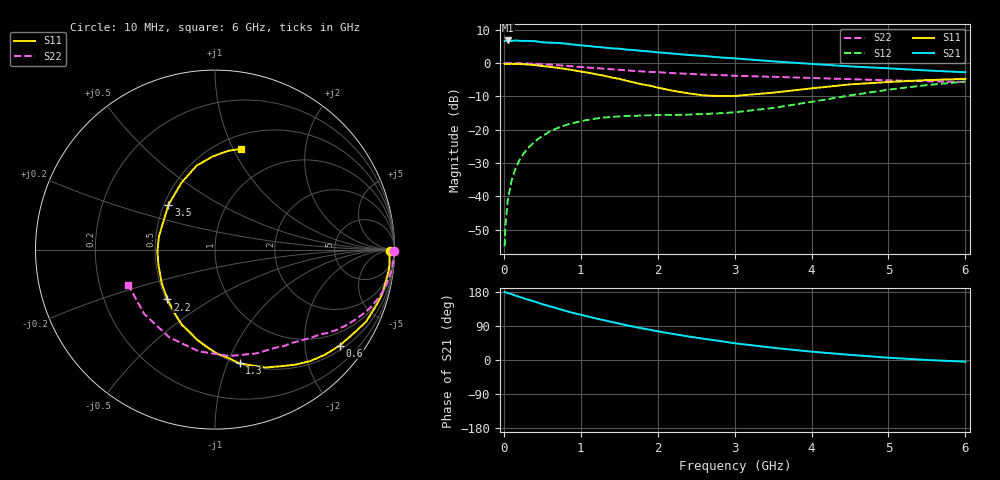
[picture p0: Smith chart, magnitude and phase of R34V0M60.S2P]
! SIEMENS Small Signal Semiconductors
! BFR181
! Si NPN RF Bipolar Junction Transistor in SOT23
! VCE = 4 V  IC = 0.6 mA
! Common Emitter S-Parameters:  May  1996
# GHz  S  MA  R  50
!  f  S11  S21  S12  S22
! GHz  MAG  ANG  MAG  ANG  MAG  ANG  MAG  ANG
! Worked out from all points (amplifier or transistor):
!   36 points, 10 MHz to 6 GHz, reference 50 ohm
!   highest |S21| = 6.8 dB at 50 MHz (marker M1)
!   |S21| within 3 dB of that: start of sweep to 1.744 GHz
!   unconditionally stable (mu >= 1): 2.286 GHz to 3.867 GHz
!   at 250 MHz: K = 0.12, MSG = 17.0 dB, |S12| = -27.4 dB
!   at 1.4 GHz: K = 0.64, MSG = 10.3 dB, |S12| = -16.2 dB
!   at 6 GHz: K = 0.91, MSG = 1.4 dB, |S12| = -5.5 dB
!   S11 on the Smith chart (normalised r, x): 10 MHz: 70, -31; 600 MHz: 0.61, -2.82; 1.3 GHz: 0.51, -1.11; 2.2 GHz: 0.51, -0.33; 3.5 GHz: 0.53, +0.30; 6 GHz: 0.64, +1.08
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0.01  0.9765 -0.6  2.136 179.7  0.0018 94.1  0.9998 -0.3
0.02  0.9707 -1.2  2.146 178.6  0.0036 93.1  0.9942 -0.7
0.05  0.9746 -3.3  2.181 176.9  0.0087 87.7  0.9988 -1.5
0.1  0.976 -6.3  2.144 173.9  0.0172 86.5  0.9971 -3.0
0.15  0.9694 -9.6  2.18 169.8  0.026 82.3  0.9941 -4.6
0.2  0.9656 -12.7  2.158 166.8  0.0344 81.7  0.9911 -6.0
0.3  0.9511 -19.0  2.151 160.1  0.051 77.1  0.9824 -9.0
0.4  0.9325 -25.6  2.131 154.3  0.0664 72.4  0.9735 -11.9
0.5  0.9016 -31.3  2.047 147.3  0.0805 68.7  0.9594 -14.7
0.6  0.8765 -37.6  2.018 141.6  0.0943 64.8  0.9454 -17.2
0.8  0.8168 -49.5  1.956 129.8  0.1174 57.7  0.9111 -22.2
1.1  0.7152 -66.7  1.802 114.5  0.1411 49.0  0.8558 -28.5
1.3  0.6485 -77.8  1.71 105.1  0.1524 44.5  0.8232 -32.1
1.5  0.5791 -88.9  1.641 96.2  0.1587 41.1  0.7913 -35.3
1.8  0.4781 -107.5  1.52 83.4  0.1642 38.0  0.7482 -39.5
2.2  0.3838 -133.6  1.387 68.7  0.167 37.0  0.7065 -45.2
2.6  0.327 -164.3  1.276 56.0  0.1725 39.5  0.6714 -50.8
3  0.321 166.8  1.176 44.2  0.1827 43.8  0.6448 -57.6
3.5  0.36 136.1  1.061 32.3  0.2122 48.9  0.6224 -68.4
4.5  0.479 102.3  0.891 13.6  0.3273 49.5  0.5741 -99.1
5.5  0.5553 82.4  0.774 0.1  0.4672 37.0  0.533 -137.8
6  0.58 75.3  0.728 -4.5  0.528 28.5  0.5215 -158.0
